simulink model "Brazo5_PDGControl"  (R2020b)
settings: Solver=VariableStepAuto  StartTime=0.0  StopTime=10.0  RelTol=1e-3
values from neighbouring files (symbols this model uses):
  b = 0.02    [robotSimulationWithConstraints.m]
  J = 0.01    [robotSimulationWithConstraints.m]
  K = 0.75    [robotSimulationWithConstraints.m]
  L = 1.1*10^-3    (= 0.0011)    [robotSimulationWithConstraints.m]
  qd = q    [robotSimulationWithConstraints.m]
  R = 5.2    [robotSimulationWithConstraints.m]
undefined symbols (not defined in the file or in its folder): deg, kg, m, N, rad, s, X, Y, Z
libraries: sm_lib x59, nesl_utility x16, robotmaniplib x1
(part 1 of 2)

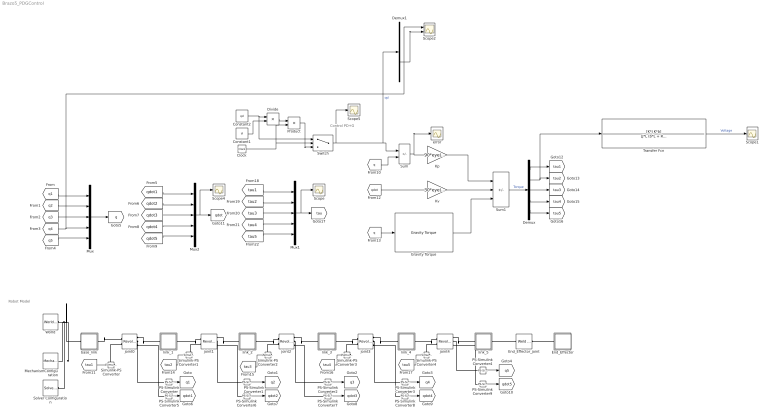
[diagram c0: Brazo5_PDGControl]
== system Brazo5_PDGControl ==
  note: Robot Model
  note: Control PD+G
  Clock : Clock
  Constant1 : Constant  Value=tf
  Constant2 : Constant  Value=qd
  Demux : Demux  Outputs=5
  Demux1 : Demux  Outputs=5
  Divide : Product  Inputs=*/
  End_Effector : Subsystem
  End_Effector_joint : sm_lib/Joints/Weld Joint  JointMode=Normal  SenseConstraintForce=off  SenseConstraintForceX=off  SenseConstraintForceY=off  SenseConstraintForceZ=off  SenseConstraintTorque=off  SenseConstraintTorqueX=off  SenseConstraintTorqueY=off  SenseConstraintTorqueZ=off  SenseTotalForce=off  SenseTotalForceX=off  SenseTotalForceY=off  SenseTotalForceZ=off  SenseTotalTorque=off  SenseTotalTorqueX=off  SenseTotalTorqueY=off  SenseTotalTorqueZ=off  CompositeWrenchDir=FollowerOnBase  CompositeWrenchFrame=BaseFrame
  Gravity Torque : robotmaniplib/Gravity Torque  RigidBodyTree=robot  SimulateUsing=Interpreted execution
  Kp : Gain  Gain=90*eye(5)  Multiplication=Matrix(K*u) (u vector)
  Kv : Gain  Gain=30*eye(5)  Multiplication=Matrix(K*u) (u vector)
  MechanismConfiguration : sm_lib/Utilities/Mechanism Configuration  UniformGravity=Constant  GravityVector=[0 0 -9.80665]  GravityVectorUnits=m/s^2  GravityUnits=m/s^2  LinearizationDelta=0.001  JointModeTransitionNonlinearIterations=2
  Mux : Mux  Inputs=5
  Mux1 : Mux  Inputs=5
  Mux2 : Mux  Inputs=5
  PS-Simulink Converter{,1..9} (10 alike) : nesl_utility/PS-Simulink Converter  PhysicalDomain=network_engine_domain  SubClassName=ps_output  LeftPortType=input  RightPortType=output  PseudoPeriodic=off  Frequencies=[]  Unit=inherit  AffineConversion=off
  Product : Product
  Scope{,1,4..5} (4 alike) : Scope
  Scope2 : Scope  NumInputPorts=2
  Simulink-PS Converter{,1..4} (5 alike) : nesl_utility/Simulink-PS Converter  PhysicalDomain=network_engine_domain  SubClassName=ps_input  LeftPortType=input  RightPortType=output  PseudoPeriodic=off  Frequencies=[]  NoiseDistribution=none  NoiseParameters=[]  Unit=1  AffineConversion=off  FilteringAndDerivatives=provide  SimscapeFilterOrder=1  InputFilterTimeConstant=0.001  UdotUserProvided=0
  Solver Configuration : nesl_utility/Solver Configuration  PhysicalDomain=network_engine_domain  SubClassName=solver  LeftPortType=input  RightPortType=generic  Tones=[]  Harmonics=[]  SimulateNoise=off  Profile=off  UseLocalSampling=off  EnableSwitchedLinearOptims=on  FrequencyDomain=off  UseCCode=off  RelTol=0.001  AbsTol=1e-06  MinStep=1e-09  ToWorkspace=off  RevertToSquareIcSolve=off  NumHomotopyIterations=100  PhasorMode=off  PhasorModeNumHarmonics=1  DoDC=off  ResidualTolerance=1e-09  UseLocalSolver=off  LocalSolverChoice=NE_BACKWARD_EULER_ADVANCER  LocalSolverSampleTime=0.001  DoFixedCost=off  MaxNonlinIter=3  MaxModeIter=2  ComputeImpulses=off  ImpulseIterations=2  LinearAlgebra=auto  EquationFormulation=NE_TIME_EF  DelaysMemoryBudget=1024  AutomaticFiltering=on  FilteringTimeConstant=0.001  PartitionStorageMethod=AS_NEEDED  PartitionMemoryBudget=1024  PartitionMethod=ROBUST
  Sum : Sum  Inputs=+-
  Sum1 : Sum  Inputs=+-+
  Switch : Switch  Criteria=u2 > Threshold  Threshold=tf
  Transfer Fcn : TransferFcn  Numerator=[K*J K*b]  Denominator=[J*L (b*L + R*J) b*R+K^2]
  World : sm_lib/Frames and Transforms/World Frame
  base_link : Subsystem
  error : Scope
  joint0 : sm_lib/Joints/Revolute Joint  JointMode=Normal  SenseConstraintForce=off  SenseConstraintForceX=off  SenseConstraintForceY=off  SenseConstraintForceZ=off  SenseConstraintTorque=off  SenseConstraintTorqueX=off  SenseConstraintTorqueY=off  SenseConstraintTorqueZ=off  SenseTotalForce=off  SenseTotalForceX=off  SenseTotalForceY=off  SenseTotalForceZ=off  SenseTotalTorque=off  SenseTotalTorqueX=off  SenseTotalTorqueY=off  SenseTotalTorqueZ=off  CompositeWrenchDir=FollowerOnBase  CompositeWrenchFrame=BaseFrame  EquilibriumPosition=0  EquilibriumPositionUnits=deg  SpringStiffness=0  SpringStiffnessUnits=N*m/deg  DampingCoefficient=0  DampingCoefficientUnits=m^2*kg/s/rad  TorqueActuationMode=InputTorque  MotionActuationMode=ComputedMotion  SensePosition=on  SenseVelocity=on  SenseAcceleration=off  SenseTorqueForce=off  SenseLowerLimitTorqueForce=off  SenseUpperLimitTorqueForce=off  LowerLimitSpecify=on  LowerLimitBound=-2.618  LowerLimitBoundUnits=rad  LowerLimitStiffness=1e4  LowerLimitStiffnessUnits=N*m/deg  LowerLimitDamping=10  LowerLimitDampingUnits=N*m/(deg/s)  LowerLimitTransitionRegionWidth=0.1  LowerLimitTransitionRegionWidthUnits=deg  UpperLimitSpecify=on  UpperLimitBound=2.618  UpperLimitBoundUnits=rad  UpperLimitStiffness=1e4  UpperLimitStiffnessUnits=N*m/deg  UpperLimitDamping=10  UpperLimitDampingUnits=N*m/(deg/s)  UpperLimitTransitionRegionWidth=0.1  UpperLimitTransitionRegionWidthUnits=deg  PositionTargetSpecify=off  PositionTargetPriority=High  PositionTargetValue=0  PositionTargetValueUnits=deg  VelocityTargetSpecify=off  VelocityTargetPriority=High  VelocityTargetValue=0  VelocityTargetValueUnits=deg/s
  joint1 : sm_lib/Joints/Revolute Joint  JointMode=Normal  SenseConstraintForce=off  SenseConstraintForceX=off  SenseConstraintForceY=off  SenseConstraintForceZ=off  SenseConstraintTorque=off  SenseConstraintTorqueX=off  SenseConstraintTorqueY=off  SenseConstraintTorqueZ=off  SenseTotalForce=off  SenseTotalForceX=off  SenseTotalForceY=off  SenseTotalForceZ=off  SenseTotalTorque=off  SenseTotalTorqueX=off  SenseTotalTorqueY=off  SenseTotalTorqueZ=off  CompositeWrenchDir=FollowerOnBase  CompositeWrenchFrame=BaseFrame  EquilibriumPosition=0  EquilibriumPositionUnits=deg  SpringStiffness=0  SpringStiffnessUnits=N*m/deg  DampingCoefficient=0  DampingCoefficientUnits=m^2*kg/s/rad  TorqueActuationMode=InputTorque  MotionActuationMode=ComputedMotion  SensePosition=on  SenseVelocity=on  SenseAcceleration=off  SenseTorqueForce=off  SenseLowerLimitTorqueForce=off  SenseUpperLimitTorqueForce=off  LowerLimitSpecify=on  LowerLimitBound=-0.5236  LowerLimitBoundUnits=rad  LowerLimitStiffness=1e4  LowerLimitStiffnessUnits=N*m/deg  LowerLimitDamping=10  LowerLimitDampingUnits=N*m/(deg/s)  LowerLimitTransitionRegionWidth=0.1  LowerLimitTransitionRegionWidthUnits=deg  UpperLimitSpecify=on  UpperLimitBound=1.7453  UpperLimitBoundUnits=rad  UpperLimitStiffness=1e4  UpperLimitStiffnessUnits=N*m/deg  UpperLimitDamping=10  UpperLimitDampingUnits=N*m/(deg/s)  UpperLimitTransitionRegionWidth=0.1  UpperLimitTransitionRegionWidthUnits=deg  PositionTargetSpecify=off  PositionTargetPriority=High  PositionTargetValue=0  PositionTargetValueUnits=deg  VelocityTargetSpecify=off  VelocityTargetPriority=High  VelocityTargetValue=0  VelocityTargetValueUnits=deg/s
  joint2 : sm_lib/Joints/Revolute Joint  JointMode=Normal  SenseConstraintForce=off  SenseConstraintForceX=off  SenseConstraintForceY=off  SenseConstraintForceZ=off  SenseConstraintTorque=off  SenseConstraintTorqueX=off  SenseConstraintTorqueY=off  SenseConstraintTorqueZ=off  SenseTotalForce=off  SenseTotalForceX=off  SenseTotalForceY=off  SenseTotalForceZ=off  SenseTotalTorque=off  SenseTotalTorqueX=off  SenseTotalTorqueY=off  SenseTotalTorqueZ=off  CompositeWrenchDir=FollowerOnBase  CompositeWrenchFrame=BaseFrame  EquilibriumPosition=0  EquilibriumPositionUnits=deg  SpringStiffness=0  SpringStiffnessUnits=N*m/deg  DampingCoefficient=0  DampingCoefficientUnits=m^2*kg/s/rad  TorqueActuationMode=InputTorque  MotionActuationMode=ComputedMotion  SensePosition=on  SenseVelocity=on  SenseAcceleration=off  SenseTorqueForce=off  SenseLowerLimitTorqueForce=off  SenseUpperLimitTorqueForce=off  LowerLimitSpecify=on  LowerLimitBound=-0.9599  LowerLimitBoundUnits=rad  LowerLimitStiffness=1e4  LowerLimitStiffnessUnits=N*m/deg  LowerLimitDamping=10  LowerLimitDampingUnits=N*m/(deg/s)  LowerLimitTransitionRegionWidth=0.1  LowerLimitTransitionRegionWidthUnits=deg  UpperLimitSpecify=on  UpperLimitBound=0.9599  UpperLimitBoundUnits=rad  UpperLimitStiffness=1e4  UpperLimitStiffnessUnits=N*m/deg  UpperLimitDamping=10  UpperLimitDampingUnits=N*m/(deg/s)  UpperLimitTransitionRegionWidth=0.1  UpperLimitTransitionRegionWidthUnits=deg  PositionTargetSpecify=off  PositionTargetPriority=High  PositionTargetValue=0  PositionTargetValueUnits=deg  VelocityTargetSpecify=off  VelocityTargetPriority=High  VelocityTargetValue=0  VelocityTargetValueUnits=deg/s
  joint3 : sm_lib/Joints/Revolute Joint  JointMode=Normal  SenseConstraintForce=off  SenseConstraintForceX=off  SenseConstraintForceY=off  SenseConstraintForceZ=off  SenseConstraintTorque=off  SenseConstraintTorqueX=off  SenseConstraintTorqueY=off  SenseConstraintTorqueZ=off  SenseTotalForce=off  SenseTotalForceX=off  SenseTotalForceY=off  SenseTotalForceZ=off  SenseTotalTorque=off  SenseTotalTorqueX=off  SenseTotalTorqueY=off  SenseTotalTorqueZ=off  CompositeWrenchDir=FollowerOnBase  CompositeWrenchFrame=BaseFrame  EquilibriumPosition=0  EquilibriumPositionUnits=deg  SpringStiffness=0  SpringStiffnessUnits=N*m/deg  DampingCoefficient=0  DampingCoefficientUnits=m^2*kg/s/rad  TorqueActuationMode=InputTorque  MotionActuationMode=ComputedMotion  SensePosition=on  SenseVelocity=on  SenseAcceleration=off  SenseTorqueForce=off  SenseLowerLimitTorqueForce=off  SenseUpperLimitTorqueForce=off  LowerLimitSpecify=on  LowerLimitBound=-1.5708  LowerLimitBoundUnits=rad  LowerLimitStiffness=1e4  LowerLimitStiffnessUnits=N*m/deg  LowerLimitDamping=10  LowerLimitDampingUnits=N*m/(deg/s)  LowerLimitTransitionRegionWidth=0.1  LowerLimitTransitionRegionWidthUnits=deg  UpperLimitSpecify=on  UpperLimitBound=1.5708  UpperLimitBoundUnits=rad  UpperLimitStiffness=1e4  UpperLimitStiffnessUnits=N*m/deg  UpperLimitDamping=10  UpperLimitDampingUnits=N*m/(deg/s)  UpperLimitTransitionRegionWidth=0.1  UpperLimitTransitionRegionWidthUnits=deg  PositionTargetSpecify=off  PositionTargetPriority=High  PositionTargetValue=0  PositionTargetValueUnits=deg  VelocityTargetSpecify=off  VelocityTargetPriority=High  VelocityTargetValue=0  VelocityTargetValueUnits=deg/s
  joint4 : sm_lib/Joints/Revolute Joint  JointMode=Normal  SenseConstraintForce=off  SenseConstraintForceX=off  SenseConstraintForceY=off  SenseConstraintForceZ=off  SenseConstraintTorque=off  SenseConstraintTorqueX=off  SenseConstraintTorqueY=off  SenseConstraintTorqueZ=off  SenseTotalForce=off  SenseTotalForceX=off  SenseTotalForceY=off  SenseTotalForceZ=off  SenseTotalTorque=off  SenseTotalTorqueX=off  SenseTotalTorqueY=off  SenseTotalTorqueZ=off  CompositeWrenchDir=FollowerOnBase  CompositeWrenchFrame=BaseFrame  EquilibriumPosition=0  EquilibriumPositionUnits=deg  SpringStiffness=0  SpringStiffnessUnits=N*m/deg  DampingCoefficient=0  DampingCoefficientUnits=m^2*kg/s/rad  TorqueActuationMode=InputTorque  MotionActuationMode=ComputedMotion  SensePosition=on  SenseVelocity=on  SenseAcceleration=off  SenseTorqueForce=off  SenseLowerLimitTorqueForce=off  SenseUpperLimitTorqueForce=off  LowerLimitSpecify=off  LowerLimitBound=-90  LowerLimitBoundUnits=deg  LowerLimitStiffness=1e4  LowerLimitStiffnessUnits=N*m/deg  LowerLimitDamping=10  LowerLimitDampingUnits=N*m/(deg/s)  LowerLimitTransitionRegionWidth=0.1  LowerLimitTransitionRegionWidthUnits=deg  UpperLimitSpecify=off  UpperLimitBound=90  UpperLimitBoundUnits=deg  UpperLimitStiffness=1e4  UpperLimitStiffnessUnits=N*m/deg  UpperLimitDamping=10  UpperLimitDampingUnits=N*m/(deg/s)  UpperLimitTransitionRegionWidth=0.1  UpperLimitTransitionRegionWidthUnits=deg  PositionTargetSpecify=off  PositionTargetPriority=High  PositionTargetValue=0  PositionTargetValueUnits=deg  VelocityTargetSpecify=off  VelocityTargetPriority=High  VelocityTargetValue=0  VelocityTargetValueUnits=deg/s
  link_1 : Subsystem
  link_2 : Subsystem
  link_3 : Subsystem
  link_4 : Subsystem
  link_5 : Subsystem
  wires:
  PS-Simulink Converter/1 -> [q1]
  [q1] -> Mux/1
  PS-Simulink Converter1/1 -> [q2]
  PS-Simulink Converter2/1 -> [q3]
  PS-Simulink Converter3/1 -> [q4]
  PS-Simulink Converter4/1 -> [q5]
  [q2] -> Mux/2
  [q3] -> Mux/3
  [q4] -> Scope2/1, Mux/4
  [q5] -> Mux/5
  Mux/1 -> [q]
  PS-Simulink Converter5/1 -> [qdot1]
  PS-Simulink Converter6/1 -> [qdot2]
  PS-Simulink Converter7/1 -> [qdot3]
  PS-Simulink Converter8/1 -> [qdot4]
  PS-Simulink Converter9/1 -> [qdot5]
  [qdot3] -> Mux2/3
  [qdot2] -> Mux2/2
  [qdot5] -> Mux2/5
  Mux2/1 -> Scope4/1, [qdot]
  [qdot1] -> Mux2/1
  [qdot4] -> Mux2/4
  Switch/1 -> Demux1/1, Sum/1, Scope5/1  "qd"
  [q] -> Sum/2
  Sum/1 -> error/1, Kp/1
  [qdot] -> Kv/1
  [q] -> Gravity Torque/1
  Kv/1 -> Sum1/2
  Kp/1 -> Sum1/1
  Demux/1 -> [tau1]
  Sum1/1 -> Demux/1  "Torque"
  Demux/5 -> [tau5]
  Demux/4 -> [tau4]
  Demux/3 -> [tau3]
  [tau1] -> Simulink-PS Converter/1
  [tau2] -> Simulink-PS Converter1/1
  [tau3] -> Simulink-PS Converter2/1
  [tau4] -> Simulink-PS Converter3/1
  [tau5] -> Simulink-PS Converter4/1
  [tau4] -> Mux1/4
  [tau2] -> Mux1/2
  [tau5] -> Mux1/5
  Mux1/1 -> Scope/1, [tau]
  [tau3] -> Mux1/3
  [tau1] -> Mux1/1
  Gravity Torque/1 -> Sum1/3
  Constant1/1 -> Divide/2
  Constant2/1 -> Divide/1, Switch/1
  Divide/1 -> Product/1
  Clock/1 -> Product/2, Switch/2
  Product/1 -> Switch/3
  Demux1/4 -> Scope2/2
  Transfer Fcn/1 -> Scope1/1  "Voltage"
  Demux/2 -> Transfer Fcn/1, [tau2]
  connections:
  End_Effector/LConn1 -- End_Effector_joint/RConn1
  base_link/RConn1 -- joint0/LConn1
  joint4/RConn1 -- link_5/LConn1
  End_Effector_joint/LConn1 -- link_5/RConn1
  World/RConn1 -- MechanismConfiguration/RConn1 -- Solver Configuration/RConn1 -- base_link/LConn1
  joint0/RConn1 -- link_1/LConn1
  joint1/LConn1 -- link_1/RConn1
  joint1/RConn1 -- link_2/LConn1
  joint2/LConn1 -- link_2/RConn1
  joint2/RConn1 -- link_3/LConn1
  joint3/LConn1 -- link_3/RConn1
  joint3/RConn1 -- link_4/LConn1
  joint4/LConn1 -- link_4/RConn1
  joint0/RConn2 -- PS-Simulink Converter/LConn1
  joint1/RConn2 -- PS-Simulink Converter1/LConn1
  joint2/RConn2 -- PS-Simulink Converter2/LConn1
  joint3/RConn2 -- PS-Simulink Converter3/LConn1
  joint4/RConn2 -- PS-Simulink Converter4/LConn1
  PS-Simulink Converter5/LConn1 -- joint0/RConn3
  PS-Simulink Converter6/LConn1 -- joint1/RConn3
  joint2/RConn3 -- PS-Simulink Converter7/LConn1
  PS-Simulink Converter8/LConn1 -- joint3/RConn3
  PS-Simulink Converter9/LConn1 -- joint4/RConn3
  Simulink-PS Converter/RConn1 -- joint0/LConn2
  Simulink-PS Converter1/RConn1 -- joint1/LConn2
  Simulink-PS Converter2/RConn1 -- joint2/LConn2
  Simulink-PS Converter3/RConn1 -- joint3/LConn2
  Simulink-PS Converter4/RConn1 -- joint4/LConn2

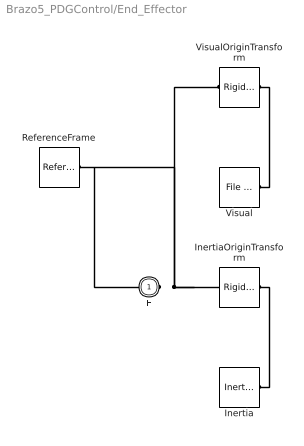
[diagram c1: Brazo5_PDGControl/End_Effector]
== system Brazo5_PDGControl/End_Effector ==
  Inertia : sm_lib/Body Elements/Inertia  InertiaType=Custom  Mass=1.4886  MassUnits=kg  CenterOfMass=[0, 0, 0]  CenterOfMassUnits=m  MomentsOfInertia=[0.00086527, 0.00086527, 0.0015073]  MomentsOfInertiaUnits=kg*m^2  ProductsOfInertia=[-1.4429e-20, -5.8421e-20, 3.3881e-21]  ProductsOfInertiaUnits=kg*m^2  GraphicType=None  MarkerShape=Inertia  MarkerSize=20  GraphicVisPropType=SimpleVisualProperties  GraphicDiffuseColor=[0.5 0.5 0.5]  GraphicSpecularColor=[0.5 0.5 0.5 1.0]  GraphicAmbientColor=[0.15 0.15 0.15 1.0]  GraphicEmissiveColor=[0.0 0.0 0.0 1.0]  GraphicShininess=75  GraphicOpacity=1.0
  InertiaOriginTransform : sm_lib/Frames and Transforms/Rigid Transform  TranslationMethod=Cartesian  TranslationStandardOffset=0  TranslationLengthUnit=m  TranslationStandardAxis=+Z  TranslationCartesianOffset=[5.5511e-17, -3.4694e-18, -0.015]  TranslationROffset=0  TranslationROffsetUnits=m  TranslationZOffset=0  TranslationZOffsetUnits=m  TranslationThetaOffset=0  TranslationThetaOffsetUnits=deg  RotationMethod=RotationSequence  RotationAngleUnits=deg  RotationStandardAxis=+Z  RotationAngle=0.0  RotationArbitraryAxis=[0 0 1]  FollAlignAxisA=+X  BaseAlignAxisA=+Y  FollAlignAxisB=+Y  BaseAlignAxisB=+Z  RotationSequenceAxes=BaseAxes  RotationSequence=XYZ  RotationSequenceAngles=[0, 0, 0]  RotationSequenceAnglesUnits=rad  RotationMatrix=[1 0 0; 0 1 0; 0 0 1]
  ReferenceFrame : sm_lib/Frames and Transforms/Reference Frame
  Visual : sm_lib/Body Elements/File Solid  ExtGeomFileName=Brazo5_SLDASM/meshes/End_Effector.STL  UnitType=Custom  ExtGeomFileUnits=m  StepReaderType=HEX  ExportConvexHullGeometry=off  InertiaType=Custom  Mass=0  MassUnits=kg  CenterOfMass=[0, 0, 0]  CenterOfMassUnits=m  MomentsOfInertia=[0, 0, 0]  MomentsOfInertiaUnits=kg*m^2  ProductsOfInertia=[0, 0, 0]  ProductsOfInertiaUnits=kg*m^2  BasedOnType=DensityFromFile  Density=1000  DensityUnits=kg/m^3  DoExposeReferenceFrame=on  SerializedFrames=<Frames/>  GraphicType=FromGeometry  MarkerShape=Sphere  MarkerSize=10  GraphicVisPropType=SimpleVisualProperties  GraphicDiffuseColor=[0.77647, 0.75686, 0.73725]  GraphicSpecularColor=[0.5 0.5 0.5 1.0]  GraphicAmbientColor=[0.15 0.15 0.15 1.0]  GraphicEmissiveColor=[0.0 0.0 0.0 1.0]  GraphicShininess=75  GraphicOpacity=1
  VisualOriginTransform : sm_lib/Frames and Transforms/Rigid Transform  TranslationMethod=Cartesian  TranslationStandardOffset=0  TranslationLengthUnit=m  TranslationStandardAxis=+Z  TranslationCartesianOffset=[0, 0, 0]  TranslationROffset=0  TranslationROffsetUnits=m  TranslationZOffset=0  TranslationZOffsetUnits=m  TranslationThetaOffset=0  TranslationThetaOffsetUnits=deg  RotationMethod=RotationSequence  RotationAngleUnits=deg  RotationStandardAxis=+Z  RotationAngle=0.0  RotationArbitraryAxis=[0 0 1]  FollAlignAxisA=+X  BaseAlignAxisA=+Y  FollAlignAxisB=+Y  BaseAlignAxisB=+Z  RotationSequenceAxes=BaseAxes  RotationSequence=XYZ  RotationSequenceAngles=[0, 0, 0]  RotationSequenceAnglesUnits=rad  RotationMatrix=[1 0 0; 0 1 0; 0 0 1]
  F : PMIOPort  Side=Left
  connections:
  Inertia/RConn1 -- InertiaOriginTransform/RConn1
  ReferenceFrame/RConn1 -- InertiaOriginTransform/LConn1 -- VisualOriginTransform/LConn1 -- F/RConn1
  Visual/RConn1 -- VisualOriginTransform/RConn1

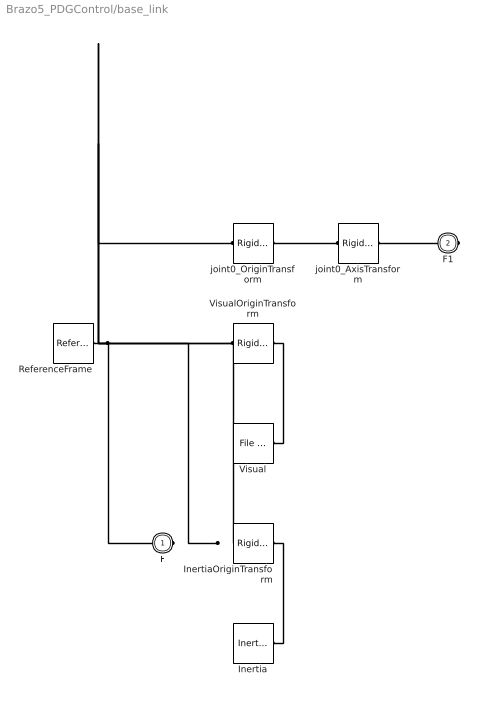
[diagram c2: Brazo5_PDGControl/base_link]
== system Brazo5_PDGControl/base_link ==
  Inertia : sm_lib/Body Elements/Inertia  InertiaType=Custom  Mass=24.7510397618277  MassUnits=kg  CenterOfMass=[0, 0, 0]  CenterOfMassUnits=m  MomentsOfInertia=[0.0874801756562005, 0.0874759059101369, 0.08538874734227481]  MomentsOfInertiaUnits=kg*m^2  ProductsOfInertia=[9.227257706190509e-08, 1.66550942408297e-07, -1.07699296841389e-07]  ProductsOfInertiaUnits=kg*m^2  GraphicType=None  MarkerShape=Inertia  MarkerSize=20  GraphicVisPropType=SimpleVisualProperties  GraphicDiffuseColor=[0.5 0.5 0.5]  GraphicSpecularColor=[0.5 0.5 0.5 1.0]  GraphicAmbientColor=[0.15 0.15 0.15 1.0]  GraphicEmissiveColor=[0.0 0.0 0.0 1.0]  GraphicShininess=75  GraphicOpacity=1.0
  InertiaOriginTransform : sm_lib/Frames and Transforms/Rigid Transform  TranslationMethod=Cartesian  TranslationStandardOffset=0  TranslationLengthUnit=m  TranslationStandardAxis=+Z  TranslationCartesianOffset=[-3.38903049823907e-08, 1.11389311641252e-06, 0.0695274745393441]  TranslationROffset=0  TranslationROffsetUnits=m  TranslationZOffset=0  TranslationZOffsetUnits=m  TranslationThetaOffset=0  TranslationThetaOffsetUnits=deg  RotationMethod=RotationSequence  RotationAngleUnits=deg  RotationStandardAxis=+Z  RotationAngle=0.0  RotationArbitraryAxis=[0 0 1]  FollAlignAxisA=+X  BaseAlignAxisA=+Y  FollAlignAxisB=+Y  BaseAlignAxisB=+Z  RotationSequenceAxes=BaseAxes  RotationSequence=XYZ  RotationSequenceAngles=[0, 0, 0]  RotationSequenceAnglesUnits=rad  RotationMatrix=[1 0 0; 0 1 0; 0 0 1]
  ReferenceFrame : sm_lib/Frames and Transforms/Reference Frame
  Visual : sm_lib/Body Elements/File Solid  ExtGeomFileName=Brazo5_SLDASM/meshes/base_link.STL  UnitType=Custom  ExtGeomFileUnits=m  StepReaderType=HEX  ExportConvexHullGeometry=off  InertiaType=Custom  Mass=0  MassUnits=kg  CenterOfMass=[0, 0, 0]  CenterOfMassUnits=m  MomentsOfInertia=[0, 0, 0]  MomentsOfInertiaUnits=kg*m^2  ProductsOfInertia=[0, 0, 0]  ProductsOfInertiaUnits=kg*m^2  BasedOnType=DensityFromFile  Density=1000  DensityUnits=kg/m^3  DoExposeReferenceFrame=on  SerializedFrames=<Frames/>  GraphicType=FromGeometry  MarkerShape=Sphere  MarkerSize=10  GraphicVisPropType=SimpleVisualProperties  GraphicDiffuseColor=[0.776470588235294, 0.756862745098039, 0.737254901960784]  GraphicSpecularColor=[0.5 0.5 0.5 1.0]  GraphicAmbientColor=[0.15 0.15 0.15 1.0]  GraphicEmissiveColor=[0.0 0.0 0.0 1.0]  GraphicShininess=75  GraphicOpacity=1
  VisualOriginTransform : sm_lib/Frames and Transforms/Rigid Transform  TranslationMethod=Cartesian  TranslationStandardOffset=0  TranslationLengthUnit=m  TranslationStandardAxis=+Z  TranslationCartesianOffset=[0, 0, 0]  TranslationROffset=0  TranslationROffsetUnits=m  TranslationZOffset=0  TranslationZOffsetUnits=m  TranslationThetaOffset=0  TranslationThetaOffsetUnits=deg  RotationMethod=RotationSequence  RotationAngleUnits=deg  RotationStandardAxis=+Z  RotationAngle=0.0  RotationArbitraryAxis=[0 0 1]  FollAlignAxisA=+X  BaseAlignAxisA=+Y  FollAlignAxisB=+Y  BaseAlignAxisB=+Z  RotationSequenceAxes=BaseAxes  RotationSequence=XYZ  RotationSequenceAngles=[0, 0, 0]  RotationSequenceAnglesUnits=rad  RotationMatrix=[1 0 0; 0 1 0; 0 0 1]
  joint0_AxisTransform : sm_lib/Frames and Transforms/Rigid Transform  TranslationMethod=Cartesian  TranslationStandardOffset=0  TranslationLengthUnit=m  TranslationStandardAxis=+Z  TranslationCartesianOffset=[0, 0, 0]  TranslationROffset=0  TranslationROffsetUnits=m  TranslationZOffset=0  TranslationZOffsetUnits=m  TranslationThetaOffset=0  TranslationThetaOffsetUnits=deg  RotationMethod=ArbitraryAxis  RotationAngleUnits=rad  RotationStandardAxis=+Z  RotationAngle=0  RotationArbitraryAxis=[1, 0, 0]  FollAlignAxisA=+X  BaseAlignAxisA=+Y  FollAlignAxisB=+Y  BaseAlignAxisB=+Z  RotationSequenceAxes=FollowerAxes  RotationSequence=XYX  RotationSequenceAngles=[0 0 0]  RotationSequenceAnglesUnits=deg  RotationMatrix=[1 0 0; 0 1 0; 0 0 1]
  joint0_OriginTransform : sm_lib/Frames and Transforms/Rigid Transform  TranslationMethod=Cartesian  TranslationStandardOffset=0  TranslationLengthUnit=m  TranslationStandardAxis=+Z  TranslationCartesianOffset=[0, 0, 0]  TranslationROffset=0  TranslationROffsetUnits=m  TranslationZOffset=0  TranslationZOffsetUnits=m  TranslationThetaOffset=0  TranslationThetaOffsetUnits=deg  RotationMethod=RotationSequence  RotationAngleUnits=deg  RotationStandardAxis=+Z  RotationAngle=0.0  RotationArbitraryAxis=[0 0 1]  FollAlignAxisA=+X  BaseAlignAxisA=+Y  FollAlignAxisB=+Y  BaseAlignAxisB=+Z  RotationSequenceAxes=BaseAxes  RotationSequence=XYZ  RotationSequenceAngles=[0, 0, 0]  RotationSequenceAnglesUnits=rad  RotationMatrix=[1 0 0; 0 1 0; 0 0 1]
  F : PMIOPort  Side=Left
  F1 : PMIOPort  Port=2  Side=Right
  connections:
  Inertia/RConn1 -- InertiaOriginTransform/RConn1
  ReferenceFrame/RConn1 -- InertiaOriginTransform/LConn1 -- VisualOriginTransform/LConn1 -- joint0_OriginTransform/LConn1 -- F/RConn1
  Visual/RConn1 -- VisualOriginTransform/RConn1
  joint0_AxisTransform/RConn1 -- F1/RConn1
  joint0_AxisTransform/LConn1 -- joint0_OriginTransform/RConn1

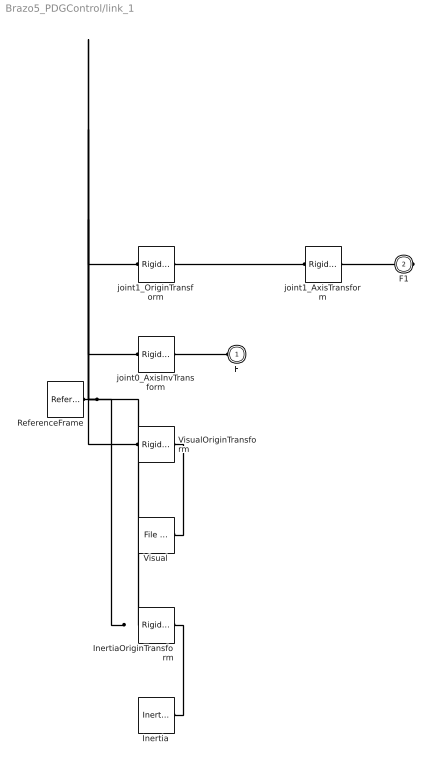
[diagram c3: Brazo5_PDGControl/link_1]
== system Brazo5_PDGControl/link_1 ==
  Inertia : sm_lib/Body Elements/Inertia  InertiaType=Custom  Mass=40.0845288402432  MassUnits=kg  CenterOfMass=[0, 0, 0]  CenterOfMassUnits=m  MomentsOfInertia=[0.14010759767158, 0.151242200998818, 0.165885928760033]  MomentsOfInertiaUnits=kg*m^2  ProductsOfInertia=[-5.20692886539246e-17, 1.32894629589073e-17, 1.5890318187219e-18]  ProductsOfInertiaUnits=kg*m^2  GraphicType=None  MarkerShape=Inertia  MarkerSize=20  GraphicVisPropType=SimpleVisualProperties  GraphicDiffuseColor=[0.5 0.5 0.5]  GraphicSpecularColor=[0.5 0.5 0.5 1.0]  GraphicAmbientColor=[0.15 0.15 0.15 1.0]  GraphicEmissiveColor=[0.0 0.0 0.0 1.0]  GraphicShininess=75  GraphicOpacity=1.0
  InertiaOriginTransform : sm_lib/Frames and Transforms/Rigid Transform  TranslationMethod=Cartesian  TranslationStandardOffset=0  TranslationLengthUnit=m  TranslationStandardAxis=+Z  TranslationCartesianOffset=[2.24939232534553e-17, 2.46845186444496e-06, 0.28325146066136]  TranslationROffset=0  TranslationROffsetUnits=m  TranslationZOffset=0  TranslationZOffsetUnits=m  TranslationThetaOffset=0  TranslationThetaOffsetUnits=deg  RotationMethod=RotationSequence  RotationAngleUnits=deg  RotationStandardAxis=+Z  RotationAngle=0.0  RotationArbitraryAxis=[0 0 1]  FollAlignAxisA=+X  BaseAlignAxisA=+Y  FollAlignAxisB=+Y  BaseAlignAxisB=+Z  RotationSequenceAxes=BaseAxes  RotationSequence=XYZ  RotationSequenceAngles=[0, 0, 0]  RotationSequenceAnglesUnits=rad  RotationMatrix=[1 0 0; 0 1 0; 0 0 1]
  ReferenceFrame : sm_lib/Frames and Transforms/Reference Frame
  Visual : sm_lib/Body Elements/File Solid  ExtGeomFileName=Brazo5_SLDASM/meshes/link_1.STL  UnitType=Custom  ExtGeomFileUnits=m  StepReaderType=HEX  ExportConvexHullGeometry=off  InertiaType=Custom  Mass=0  MassUnits=kg  CenterOfMass=[0, 0, 0]  CenterOfMassUnits=m  MomentsOfInertia=[0, 0, 0]  MomentsOfInertiaUnits=kg*m^2  ProductsOfInertia=[0, 0, 0]  ProductsOfInertiaUnits=kg*m^2  BasedOnType=DensityFromFile  Density=1000  DensityUnits=kg/m^3  DoExposeReferenceFrame=on  SerializedFrames=<Frames/>  GraphicType=FromGeometry  MarkerShape=Sphere  MarkerSize=10  GraphicVisPropType=SimpleVisualProperties  GraphicDiffuseColor=[0.776470588235294, 0.756862745098039, 0.737254901960784]  GraphicSpecularColor=[0.5 0.5 0.5 1.0]  GraphicAmbientColor=[0.15 0.15 0.15 1.0]  GraphicEmissiveColor=[0.0 0.0 0.0 1.0]  GraphicShininess=75  GraphicOpacity=1
  VisualOriginTransform : sm_lib/Frames and Transforms/Rigid Transform  TranslationMethod=Cartesian  TranslationStandardOffset=0  TranslationLengthUnit=m  TranslationStandardAxis=+Z  TranslationCartesianOffset=[0, 0, 0]  TranslationROffset=0  TranslationROffsetUnits=m  TranslationZOffset=0  TranslationZOffsetUnits=m  TranslationThetaOffset=0  TranslationThetaOffsetUnits=deg  RotationMethod=RotationSequence  RotationAngleUnits=deg  RotationStandardAxis=+Z  RotationAngle=0.0  RotationArbitraryAxis=[0 0 1]  FollAlignAxisA=+X  BaseAlignAxisA=+Y  FollAlignAxisB=+Y  BaseAlignAxisB=+Z  RotationSequenceAxes=BaseAxes  RotationSequence=XYZ  RotationSequenceAngles=[0, 0, 0]  RotationSequenceAnglesUnits=rad  RotationMatrix=[1 0 0; 0 1 0; 0 0 1]
  joint0_AxisInvTransform : sm_lib/Frames and Transforms/Rigid Transform  TranslationMethod=Cartesian  TranslationStandardOffset=0  TranslationLengthUnit=m  TranslationStandardAxis=+Z  TranslationCartesianOffset=[0, 0, 0]  TranslationROffset=0  TranslationROffsetUnits=m  TranslationZOffset=0  TranslationZOffsetUnits=m  TranslationThetaOffset=0  TranslationThetaOffsetUnits=deg  RotationMethod=ArbitraryAxis  RotationAngleUnits=rad  RotationStandardAxis=+Z  RotationAngle=0  RotationArbitraryAxis=[1, 0, 0]  FollAlignAxisA=+X  BaseAlignAxisA=+Y  FollAlignAxisB=+Y  BaseAlignAxisB=+Z  RotationSequenceAxes=FollowerAxes  RotationSequence=XYX  RotationSequenceAngles=[0 0 0]  RotationSequenceAnglesUnits=deg  RotationMatrix=[1 0 0; 0 1 0; 0 0 1]
  joint1_AxisTransform : sm_lib/Frames and Transforms/Rigid Transform  TranslationMethod=Cartesian  TranslationStandardOffset=0  TranslationLengthUnit=m  TranslationStandardAxis=+Z  TranslationCartesianOffset=[0, 0, 0]  TranslationROffset=0  TranslationROffsetUnits=m  TranslationZOffset=0  TranslationZOffsetUnits=m  TranslationThetaOffset=0  TranslationThetaOffsetUnits=deg  RotationMethod=ArbitraryAxis  RotationAngleUnits=rad  RotationStandardAxis=+Z  RotationAngle=0  RotationArbitraryAxis=[1, 0, 0]  FollAlignAxisA=+X  BaseAlignAxisA=+Y  FollAlignAxisB=+Y  BaseAlignAxisB=+Z  RotationSequenceAxes=FollowerAxes  RotationSequence=XYX  RotationSequenceAngles=[0 0 0]  RotationSequenceAnglesUnits=deg  RotationMatrix=[1 0 0; 0 1 0; 0 0 1]
  joint1_OriginTransform : sm_lib/Frames and Transforms/Rigid Transform  TranslationMethod=Cartesian  TranslationStandardOffset=0  TranslationLengthUnit=m  TranslationStandardAxis=+Z  TranslationCartesianOffset=[0, 0, 0.35051]  TranslationROffset=0  TranslationROffsetUnits=m  TranslationZOffset=0  TranslationZOffsetUnits=m  TranslationThetaOffset=0  TranslationThetaOffsetUnits=deg  RotationMethod=RotationSequence  RotationAngleUnits=deg  RotationStandardAxis=+Z  RotationAngle=0.0  RotationArbitraryAxis=[0 0 1]  FollAlignAxisA=+X  BaseAlignAxisA=+Y  FollAlignAxisB=+Y  BaseAlignAxisB=+Z  RotationSequenceAxes=BaseAxes  RotationSequence=XYZ  RotationSequenceAngles=[1.5708, 0, 1.5708]  RotationSequenceAnglesUnits=rad  RotationMatrix=[1 0 0; 0 1 0; 0 0 1]
  F : PMIOPort  Side=Left
  F1 : PMIOPort  Port=2  Side=Right
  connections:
  Inertia/RConn1 -- InertiaOriginTransform/RConn1
  ReferenceFrame/RConn1 -- InertiaOriginTransform/LConn1 -- VisualOriginTransform/LConn1 -- joint0_AxisInvTransform/LConn1 -- joint1_OriginTransform/LConn1
  Visual/RConn1 -- VisualOriginTransform/RConn1
  joint0_AxisInvTransform/RConn1 -- F/RConn1
  joint1_AxisTransform/RConn1 -- F1/RConn1
  joint1_AxisTransform/LConn1 -- joint1_OriginTransform/RConn1

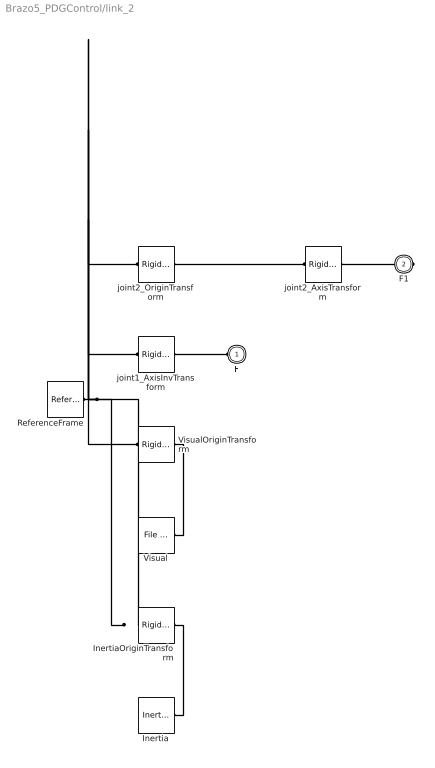
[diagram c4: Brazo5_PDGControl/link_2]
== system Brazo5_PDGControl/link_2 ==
  Inertia : sm_lib/Body Elements/Inertia  InertiaType=Custom  Mass=34.1892669715201  MassUnits=kg  CenterOfMass=[0, 0, 0]  CenterOfMassUnits=m  MomentsOfInertia=[0.100999689869813, 0.323464785078339, 0.28584252374745]  MomentsOfInertiaUnits=kg*m^2  ProductsOfInertia=[-2.19096219704951e-18, 8.5802322320121e-17, 3.73980846905113e-17]  ProductsOfInertiaUnits=kg*m^2  GraphicType=None  MarkerShape=Inertia  MarkerSize=20  GraphicVisPropType=SimpleVisualProperties  GraphicDiffuseColor=[0.5 0.5 0.5]  GraphicSpecularColor=[0.5 0.5 0.5 1.0]  GraphicAmbientColor=[0.15 0.15 0.15 1.0]  GraphicEmissiveColor=[0.0 0.0 0.0 1.0]  GraphicShininess=75  GraphicOpacity=1.0
  InertiaOriginTransform : sm_lib/Frames and Transforms/Rigid Transform  TranslationMethod=Cartesian  TranslationStandardOffset=0  TranslationLengthUnit=m  TranslationStandardAxis=+Z  TranslationCartesianOffset=[0.07391242231991781, 0, -1.2931997966502e-17]  TranslationROffset=0  TranslationROffsetUnits=m  TranslationZOffset=0  TranslationZOffsetUnits=m  TranslationThetaOffset=0  TranslationThetaOffsetUnits=deg  RotationMethod=RotationSequence  RotationAngleUnits=deg  RotationStandardAxis=+Z  RotationAngle=0.0  RotationArbitraryAxis=[0 0 1]  FollAlignAxisA=+X  BaseAlignAxisA=+Y  FollAlignAxisB=+Y  BaseAlignAxisB=+Z  RotationSequenceAxes=BaseAxes  RotationSequence=XYZ  RotationSequenceAngles=[0, 0, 0]  RotationSequenceAnglesUnits=rad  RotationMatrix=[1 0 0; 0 1 0; 0 0 1]
  ReferenceFrame : sm_lib/Frames and Transforms/Reference Frame
  Visual : sm_lib/Body Elements/File Solid  ExtGeomFileName=Brazo5_SLDASM/meshes/link_2.STL  UnitType=Custom  ExtGeomFileUnits=m  StepReaderType=HEX  ExportConvexHullGeometry=off  InertiaType=Custom  Mass=0  MassUnits=kg  CenterOfMass=[0, 0, 0]  CenterOfMassUnits=m  MomentsOfInertia=[0, 0, 0]  MomentsOfInertiaUnits=kg*m^2  ProductsOfInertia=[0, 0, 0]  ProductsOfInertiaUnits=kg*m^2  BasedOnType=DensityFromFile  Density=1000  DensityUnits=kg/m^3  DoExposeReferenceFrame=on  SerializedFrames=<Frames/>  GraphicType=FromGeometry  MarkerShape=Sphere  MarkerSize=10  GraphicVisPropType=SimpleVisualProperties  GraphicDiffuseColor=[0.776470588235294, 0.756862745098039, 0.737254901960784]  GraphicSpecularColor=[0.5 0.5 0.5 1.0]  GraphicAmbientColor=[0.15 0.15 0.15 1.0]  GraphicEmissiveColor=[0.0 0.0 0.0 1.0]  GraphicShininess=75  GraphicOpacity=1
  VisualOriginTransform : sm_lib/Frames and Transforms/Rigid Transform  TranslationMethod=Cartesian  TranslationStandardOffset=0  TranslationLengthUnit=m  TranslationStandardAxis=+Z  TranslationCartesianOffset=[0, 0, 0]  TranslationROffset=0  TranslationROffsetUnits=m  TranslationZOffset=0  TranslationZOffsetUnits=m  TranslationThetaOffset=0  TranslationThetaOffsetUnits=deg  RotationMethod=RotationSequence  RotationAngleUnits=deg  RotationStandardAxis=+Z  RotationAngle=0.0  RotationArbitraryAxis=[0 0 1]  FollAlignAxisA=+X  BaseAlignAxisA=+Y  FollAlignAxisB=+Y  BaseAlignAxisB=+Z  RotationSequenceAxes=BaseAxes  RotationSequence=XYZ  RotationSequenceAngles=[0, 0, 0]  RotationSequenceAnglesUnits=rad  RotationMatrix=[1 0 0; 0 1 0; 0 0 1]
  joint1_AxisInvTransform : sm_lib/Frames and Transforms/Rigid Transform  TranslationMethod=Cartesian  TranslationStandardOffset=0  TranslationLengthUnit=m  TranslationStandardAxis=+Z  TranslationCartesianOffset=[0, 0, 0]  TranslationROffset=0  TranslationROffsetUnits=m  TranslationZOffset=0  TranslationZOffsetUnits=m  TranslationThetaOffset=0  TranslationThetaOffsetUnits=deg  RotationMethod=ArbitraryAxis  RotationAngleUnits=rad  RotationStandardAxis=+Z  RotationAngle=0  RotationArbitraryAxis=[1, 0, 0]  FollAlignAxisA=+X  BaseAlignAxisA=+Y  FollAlignAxisB=+Y  BaseAlignAxisB=+Z  RotationSequenceAxes=FollowerAxes  RotationSequence=XYX  RotationSequenceAngles=[0 0 0]  RotationSequenceAnglesUnits=deg  RotationMatrix=[1 0 0; 0 1 0; 0 0 1]
  joint2_AxisTransform : sm_lib/Frames and Transforms/Rigid Transform  TranslationMethod=Cartesian  TranslationStandardOffset=0  TranslationLengthUnit=m  TranslationStandardAxis=+Z  TranslationCartesianOffset=[0, 0, 0]  TranslationROffset=0  TranslationROffsetUnits=m  TranslationZOffset=0  TranslationZOffsetUnits=m  TranslationThetaOffset=0  TranslationThetaOffsetUnits=deg  RotationMethod=ArbitraryAxis  RotationAngleUnits=rad  RotationStandardAxis=+Z  RotationAngle=0  RotationArbitraryAxis=[1, 0, 0]  FollAlignAxisA=+X  BaseAlignAxisA=+Y  FollAlignAxisB=+Y  BaseAlignAxisB=+Z  RotationSequenceAxes=FollowerAxes  RotationSequence=XYX  RotationSequenceAngles=[0 0 0]  RotationSequenceAnglesUnits=deg  RotationMatrix=[1 0 0; 0 1 0; 0 0 1]
  joint2_OriginTransform : sm_lib/Frames and Transforms/Rigid Transform  TranslationMethod=Cartesian  TranslationStandardOffset=0  TranslationLengthUnit=m  TranslationStandardAxis=+Z  TranslationCartesianOffset=[0.25, 0, 0]  TranslationROffset=0  TranslationROffsetUnits=m  TranslationZOffset=0  TranslationZOffsetUnits=m  TranslationThetaOffset=0  TranslationThetaOffsetUnits=deg  RotationMethod=RotationSequence  RotationAngleUnits=deg  RotationStandardAxis=+Z  RotationAngle=0.0  RotationArbitraryAxis=[0 0 1]  FollAlignAxisA=+X  BaseAlignAxisA=+Y  FollAlignAxisB=+Y  BaseAlignAxisB=+Z  RotationSequenceAxes=BaseAxes  RotationSequence=XYZ  RotationSequenceAngles=[0, 0, 0]  RotationSequenceAnglesUnits=rad  RotationMatrix=[1 0 0; 0 1 0; 0 0 1]
  F : PMIOPort  Side=Left
  F1 : PMIOPort  Port=2  Side=Right
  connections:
  Inertia/RConn1 -- InertiaOriginTransform/RConn1
  ReferenceFrame/RConn1 -- InertiaOriginTransform/LConn1 -- VisualOriginTransform/LConn1 -- joint1_AxisInvTransform/LConn1 -- joint2_OriginTransform/LConn1
  Visual/RConn1 -- VisualOriginTransform/RConn1
  joint1_AxisInvTransform/RConn1 -- F/RConn1
  joint2_AxisTransform/RConn1 -- F1/RConn1
  joint2_AxisTransform/LConn1 -- joint2_OriginTransform/RConn1

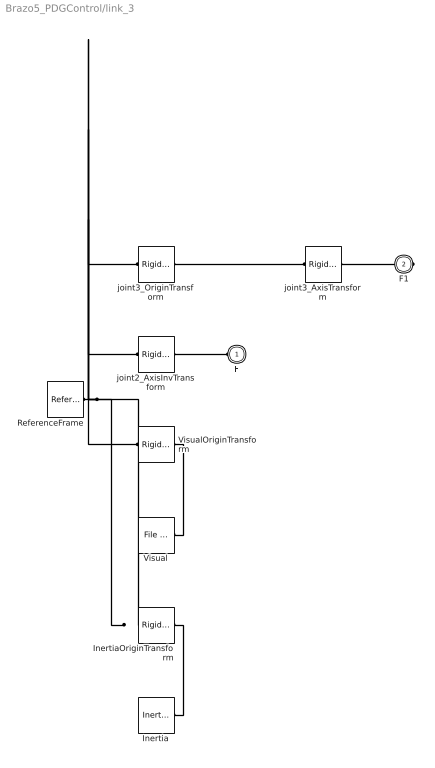
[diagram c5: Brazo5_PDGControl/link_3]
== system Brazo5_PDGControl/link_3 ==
  Inertia : sm_lib/Body Elements/Inertia  InertiaType=Custom  Mass=13.9460998385185  MassUnits=kg  CenterOfMass=[0, 0, 0]  CenterOfMassUnits=m  MomentsOfInertia=[0.026465483583986, 0.0628137115265308, 0.0543358776965413]  MomentsOfInertiaUnits=kg*m^2  ProductsOfInertia=[-5.14627121152742e-19, 1.96375333381757e-17, 6.41551043751981e-18]  ProductsOfInertiaUnits=kg*m^2  GraphicType=None  MarkerShape=Inertia  MarkerSize=20  GraphicVisPropType=SimpleVisualProperties  GraphicDiffuseColor=[0.5 0.5 0.5]  GraphicSpecularColor=[0.5 0.5 0.5 1.0]  GraphicAmbientColor=[0.15 0.15 0.15 1.0]  GraphicEmissiveColor=[0.0 0.0 0.0 1.0]  GraphicShininess=75  GraphicOpacity=1.0
  InertiaOriginTransform : sm_lib/Frames and Transforms/Rigid Transform  TranslationMethod=Cartesian  TranslationStandardOffset=0  TranslationLengthUnit=m  TranslationStandardAxis=+Z  TranslationCartesianOffset=[0.0538405076409555, 0, -2.89254125393904e-17]  TranslationROffset=0  TranslationROffsetUnits=m  TranslationZOffset=0  TranslationZOffsetUnits=m  TranslationThetaOffset=0  TranslationThetaOffsetUnits=deg  RotationMethod=RotationSequence  RotationAngleUnits=deg  RotationStandardAxis=+Z  RotationAngle=0.0  RotationArbitraryAxis=[0 0 1]  FollAlignAxisA=+X  BaseAlignAxisA=+Y  FollAlignAxisB=+Y  BaseAlignAxisB=+Z  RotationSequenceAxes=BaseAxes  RotationSequence=XYZ  RotationSequenceAngles=[0, 0, 0]  RotationSequenceAnglesUnits=rad  RotationMatrix=[1 0 0; 0 1 0; 0 0 1]
  ReferenceFrame : sm_lib/Frames and Transforms/Reference Frame
  Visual : sm_lib/Body Elements/File Solid  ExtGeomFileName=Brazo5_SLDASM/meshes/link_3.STL  UnitType=Custom  ExtGeomFileUnits=m  StepReaderType=HEX  ExportConvexHullGeometry=off  InertiaType=Custom  Mass=0  MassUnits=kg  CenterOfMass=[0, 0, 0]  CenterOfMassUnits=m  MomentsOfInertia=[0, 0, 0]  MomentsOfInertiaUnits=kg*m^2  ProductsOfInertia=[0, 0, 0]  ProductsOfInertiaUnits=kg*m^2  BasedOnType=DensityFromFile  Density=1000  DensityUnits=kg/m^3  DoExposeReferenceFrame=on  SerializedFrames=<Frames/>  GraphicType=FromGeometry  MarkerShape=Sphere  MarkerSize=10  GraphicVisPropType=SimpleVisualProperties  GraphicDiffuseColor=[0.776470588235294, 0.756862745098039, 0.737254901960784]  GraphicSpecularColor=[0.5 0.5 0.5 1.0]  GraphicAmbientColor=[0.15 0.15 0.15 1.0]  GraphicEmissiveColor=[0.0 0.0 0.0 1.0]  GraphicShininess=75  GraphicOpacity=1
  VisualOriginTransform : sm_lib/Frames and Transforms/Rigid Transform  TranslationMethod=Cartesian  TranslationStandardOffset=0  TranslationLengthUnit=m  TranslationStandardAxis=+Z  TranslationCartesianOffset=[0, 0, 0]  TranslationROffset=0  TranslationROffsetUnits=m  TranslationZOffset=0  TranslationZOffsetUnits=m  TranslationThetaOffset=0  TranslationThetaOffsetUnits=deg  RotationMethod=RotationSequence  RotationAngleUnits=deg  RotationStandardAxis=+Z  RotationAngle=0.0  RotationArbitraryAxis=[0 0 1]  FollAlignAxisA=+X  BaseAlignAxisA=+Y  FollAlignAxisB=+Y  BaseAlignAxisB=+Z  RotationSequenceAxes=BaseAxes  RotationSequence=XYZ  RotationSequenceAngles=[0, 0, 0]  RotationSequenceAnglesUnits=rad  RotationMatrix=[1 0 0; 0 1 0; 0 0 1]
  joint2_AxisInvTransform : sm_lib/Frames and Transforms/Rigid Transform  TranslationMethod=Cartesian  TranslationStandardOffset=0  TranslationLengthUnit=m  TranslationStandardAxis=+Z  TranslationCartesianOffset=[0, 0, 0]  TranslationROffset=0  TranslationROffsetUnits=m  TranslationZOffset=0  TranslationZOffsetUnits=m  TranslationThetaOffset=0  TranslationThetaOffsetUnits=deg  RotationMethod=ArbitraryAxis  RotationAngleUnits=rad  RotationStandardAxis=+Z  RotationAngle=0  RotationArbitraryAxis=[1, 0, 0]  FollAlignAxisA=+X  BaseAlignAxisA=+Y  FollAlignAxisB=+Y  BaseAlignAxisB=+Z  RotationSequenceAxes=FollowerAxes  RotationSequence=XYX  RotationSequenceAngles=[0 0 0]  RotationSequenceAnglesUnits=deg  RotationMatrix=[1 0 0; 0 1 0; 0 0 1]
  joint3_AxisTransform : sm_lib/Frames and Transforms/Rigid Transform  TranslationMethod=Cartesian  TranslationStandardOffset=0  TranslationLengthUnit=m  TranslationStandardAxis=+Z  TranslationCartesianOffset=[0, 0, 0]  TranslationROffset=0  TranslationROffsetUnits=m  TranslationZOffset=0  TranslationZOffsetUnits=m  TranslationThetaOffset=0  TranslationThetaOffsetUnits=deg  RotationMethod=ArbitraryAxis  RotationAngleUnits=rad  RotationStandardAxis=+Z  RotationAngle=0  RotationArbitraryAxis=[1, 0, 0]  FollAlignAxisA=+X  BaseAlignAxisA=+Y  FollAlignAxisB=+Y  BaseAlignAxisB=+Z  RotationSequenceAxes=FollowerAxes  RotationSequence=XYX  RotationSequenceAngles=[0 0 0]  RotationSequenceAnglesUnits=deg  RotationMatrix=[1 0 0; 0 1 0; 0 0 1]
  joint3_OriginTransform : sm_lib/Frames and Transforms/Rigid Transform  TranslationMethod=Cartesian  TranslationStandardOffset=0  TranslationLengthUnit=m  TranslationStandardAxis=+Z  TranslationCartesianOffset=[0.16, 0, 0]  TranslationROffset=0  TranslationROffsetUnits=m  TranslationZOffset=0  TranslationZOffsetUnits=m  TranslationThetaOffset=0  TranslationThetaOffsetUnits=deg  RotationMethod=RotationSequence  RotationAngleUnits=deg  RotationStandardAxis=+Z  RotationAngle=0.0  RotationArbitraryAxis=[0 0 1]  FollAlignAxisA=+X  BaseAlignAxisA=+Y  FollAlignAxisB=+Y  BaseAlignAxisB=+Z  RotationSequenceAxes=BaseAxes  RotationSequence=XYZ  RotationSequenceAngles=[0, 0, 0]  RotationSequenceAnglesUnits=rad  RotationMatrix=[1 0 0; 0 1 0; 0 0 1]
  F : PMIOPort  Side=Left
  F1 : PMIOPort  Port=2  Side=Right
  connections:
  Inertia/RConn1 -- InertiaOriginTransform/RConn1
  ReferenceFrame/RConn1 -- InertiaOriginTransform/LConn1 -- VisualOriginTransform/LConn1 -- joint2_AxisInvTransform/LConn1 -- joint3_OriginTransform/LConn1
  Visual/RConn1 -- VisualOriginTransform/RConn1
  joint2_AxisInvTransform/RConn1 -- F/RConn1
  joint3_AxisTransform/RConn1 -- F1/RConn1
  joint3_AxisTransform/LConn1 -- joint3_OriginTransform/RConn1

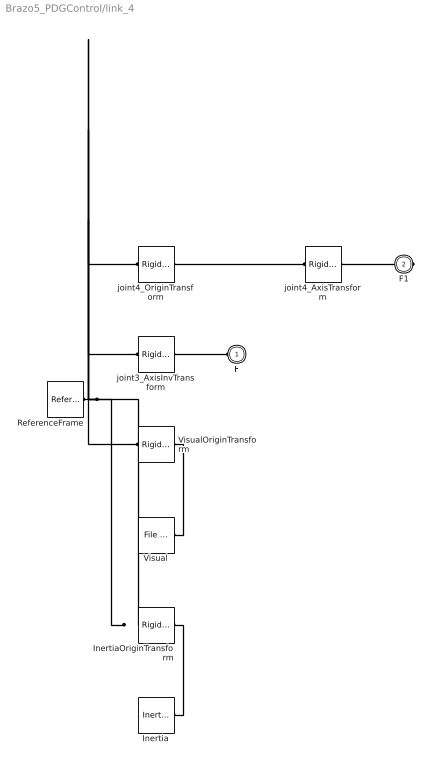
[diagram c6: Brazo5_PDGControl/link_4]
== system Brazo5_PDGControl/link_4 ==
  Inertia : sm_lib/Body Elements/Inertia  InertiaType=Custom  Mass=2.62582123658694  MassUnits=kg  CenterOfMass=[0, 0, 0]  CenterOfMassUnits=m  MomentsOfInertia=[0.00197083600155281, 0.00325865261538323, 0.00214733918833594]  MomentsOfInertiaUnits=kg*m^2  ProductsOfInertia=[-1.26269021628898e-19, -3.10811231220588e-19, 2.23060660101183e-20]  ProductsOfInertiaUnits=kg*m^2  GraphicType=None  MarkerShape=Inertia  MarkerSize=20  GraphicVisPropType=SimpleVisualProperties  GraphicDiffuseColor=[0.5 0.5 0.5]  GraphicSpecularColor=[0.5 0.5 0.5 1.0]  GraphicAmbientColor=[0.15 0.15 0.15 1.0]  GraphicEmissiveColor=[0.0 0.0 0.0 1.0]  GraphicShininess=75  GraphicOpacity=1.0
  InertiaOriginTransform : sm_lib/Frames and Transforms/Rigid Transform  TranslationMethod=Cartesian  TranslationStandardOffset=0  TranslationLengthUnit=m  TranslationStandardAxis=+Z  TranslationCartesianOffset=[0.0260264378448915, -5.55111512312578e-17, 3.20676455869593e-17]  TranslationROffset=0  TranslationROffsetUnits=m  TranslationZOffset=0  TranslationZOffsetUnits=m  TranslationThetaOffset=0  TranslationThetaOffsetUnits=deg  RotationMethod=RotationSequence  RotationAngleUnits=deg  RotationStandardAxis=+Z  RotationAngle=0.0  RotationArbitraryAxis=[0 0 1]  FollAlignAxisA=+X  BaseAlignAxisA=+Y  FollAlignAxisB=+Y  BaseAlignAxisB=+Z  RotationSequenceAxes=BaseAxes  RotationSequence=XYZ  RotationSequenceAngles=[0, 0, 0]  RotationSequenceAnglesUnits=rad  RotationMatrix=[1 0 0; 0 1 0; 0 0 1]
  ReferenceFrame : sm_lib/Frames and Transforms/Reference Frame
  Visual : sm_lib/Body Elements/File Solid  ExtGeomFileName=Brazo5_SLDASM/meshes/link_4.STL  UnitType=Custom  ExtGeomFileUnits=m  StepReaderType=HEX  ExportConvexHullGeometry=off  InertiaType=Custom  Mass=0  MassUnits=kg  CenterOfMass=[0, 0, 0]  CenterOfMassUnits=m  MomentsOfInertia=[0, 0, 0]  MomentsOfInertiaUnits=kg*m^2  ProductsOfInertia=[0, 0, 0]  ProductsOfInertiaUnits=kg*m^2  BasedOnType=DensityFromFile  Density=1000  DensityUnits=kg/m^3  DoExposeReferenceFrame=on  SerializedFrames=<Frames/>  GraphicType=FromGeometry  MarkerShape=Sphere  MarkerSize=10  GraphicVisPropType=SimpleVisualProperties  GraphicDiffuseColor=[0.776470588235294, 0.756862745098039, 0.737254901960784]  GraphicSpecularColor=[0.5 0.5 0.5 1.0]  GraphicAmbientColor=[0.15 0.15 0.15 1.0]  GraphicEmissiveColor=[0.0 0.0 0.0 1.0]  GraphicShininess=75  GraphicOpacity=1
  VisualOriginTransform : sm_lib/Frames and Transforms/Rigid Transform  TranslationMethod=Cartesian  TranslationStandardOffset=0  TranslationLengthUnit=m  TranslationStandardAxis=+Z  TranslationCartesianOffset=[0, 0, 0]  TranslationROffset=0  TranslationROffsetUnits=m  TranslationZOffset=0  TranslationZOffsetUnits=m  TranslationThetaOffset=0  TranslationThetaOffsetUnits=deg  RotationMethod=RotationSequence  RotationAngleUnits=deg  RotationStandardAxis=+Z  RotationAngle=0.0  RotationArbitraryAxis=[0 0 1]  FollAlignAxisA=+X  BaseAlignAxisA=+Y  FollAlignAxisB=+Y  BaseAlignAxisB=+Z  RotationSequenceAxes=BaseAxes  RotationSequence=XYZ  RotationSequenceAngles=[0, 0, 0]  RotationSequenceAnglesUnits=rad  RotationMatrix=[1 0 0; 0 1 0; 0 0 1]
  joint3_AxisInvTransform : sm_lib/Frames and Transforms/Rigid Transform  TranslationMethod=Cartesian  TranslationStandardOffset=0  TranslationLengthUnit=m  TranslationStandardAxis=+Z  TranslationCartesianOffset=[0, 0, 0]  TranslationROffset=0  TranslationROffsetUnits=m  TranslationZOffset=0  TranslationZOffsetUnits=m  TranslationThetaOffset=0  TranslationThetaOffsetUnits=deg  RotationMethod=ArbitraryAxis  RotationAngleUnits=rad  RotationStandardAxis=+Z  RotationAngle=0  RotationArbitraryAxis=[1, 0, 0]  FollAlignAxisA=+X  BaseAlignAxisA=+Y  FollAlignAxisB=+Y  BaseAlignAxisB=+Z  RotationSequenceAxes=FollowerAxes  RotationSequence=XYX  RotationSequenceAngles=[0 0 0]  RotationSequenceAnglesUnits=deg  RotationMatrix=[1 0 0; 0 1 0; 0 0 1]
  joint4_AxisTransform : sm_lib/Frames and Transforms/Rigid Transform  TranslationMethod=Cartesian  TranslationStandardOffset=0  TranslationLengthUnit=m  TranslationStandardAxis=+Z  TranslationCartesianOffset=[0, 0, 0]  TranslationROffset=0  TranslationROffsetUnits=m  TranslationZOffset=0  TranslationZOffsetUnits=m  TranslationThetaOffset=0  TranslationThetaOffsetUnits=deg  RotationMethod=ArbitraryAxis  RotationAngleUnits=rad  RotationStandardAxis=+Z  RotationAngle=0  RotationArbitraryAxis=[1, 0, 0]  FollAlignAxisA=+X  BaseAlignAxisA=+Y  FollAlignAxisB=+Y  BaseAlignAxisB=+Z  RotationSequenceAxes=FollowerAxes  RotationSequence=XYX  RotationSequenceAngles=[0 0 0]  RotationSequenceAnglesUnits=deg  RotationMatrix=[1 0 0; 0 1 0; 0 0 1]
  joint4_OriginTransform : sm_lib/Frames and Transforms/Rigid Transform  TranslationMethod=Cartesian  TranslationStandardOffset=0  TranslationLengthUnit=m  TranslationStandardAxis=+Z  TranslationCartesianOffset=[0, 0, 0]  TranslationROffset=0  TranslationROffsetUnits=m  TranslationZOffset=0  TranslationZOffsetUnits=m  TranslationThetaOffset=0  TranslationThetaOffsetUnits=deg  RotationMethod=RotationSequence  RotationAngleUnits=deg  RotationStandardAxis=+Z  RotationAngle=0.0  RotationArbitraryAxis=[0 0 1]  FollAlignAxisA=+X  BaseAlignAxisA=+Y  FollAlignAxisB=+Y  BaseAlignAxisB=+Z  RotationSequenceAxes=BaseAxes  RotationSequence=XYZ  RotationSequenceAngles=[1.5708, 0, 1.5708]  RotationSequenceAnglesUnits=rad  RotationMatrix=[1 0 0; 0 1 0; 0 0 1]
  F : PMIOPort  Side=Left
  F1 : PMIOPort  Port=2  Side=Right
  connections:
  Inertia/RConn1 -- InertiaOriginTransform/RConn1
  ReferenceFrame/RConn1 -- InertiaOriginTransform/LConn1 -- VisualOriginTransform/LConn1 -- joint3_AxisInvTransform/LConn1 -- joint4_OriginTransform/LConn1
  Visual/RConn1 -- VisualOriginTransform/RConn1
  joint3_AxisInvTransform/RConn1 -- F/RConn1
  joint4_AxisTransform/RConn1 -- F1/RConn1
  joint4_AxisTransform/LConn1 -- joint4_OriginTransform/RConn1
